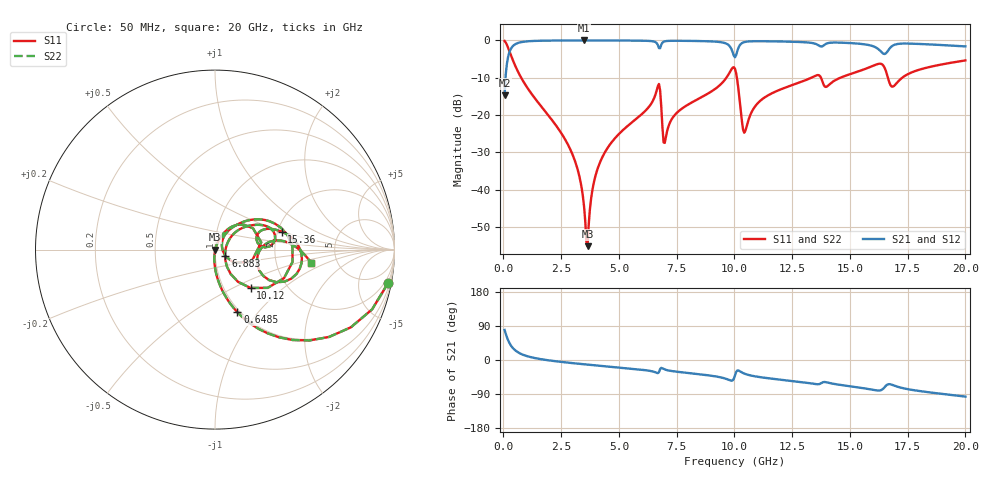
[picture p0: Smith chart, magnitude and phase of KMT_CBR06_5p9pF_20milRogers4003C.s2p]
! Data measured by Modelithics Inc. support@modelithics.com 813-866-6335
! KEMET CBR0603 5.9pF, Pad Width= 0.851mm, Pad Length= 0.64mm, Pad Gap= 0.62mm, 20mil Rogers 4003C substrate Data, January 2022
# hz S ma R 50
! 2 Port Network Data from SP1.SP block
! freq  magS11  angS11  magS21  angS21  magS12  angS12  magS22  angS22
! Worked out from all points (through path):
!   401 points, 50 MHz to 20 GHz, reference 50 ohm
!   highest |S21| = -0.01 dB at 3.491 GHz (marker M1); lowest = -14.7 dB at 50 MHz (marker M2)
!   group delay of S21, straight-line fit = 14.9 ps
!   lowest |S11| = -55.1 dB at 3.641 GHz (marker M3), VSWR 1.00, Z = 50.2 + j0.0524 ohm
!   |S11| at or under -10 dB: 767.8 MHz to 9.652 GHz (8.884 GHz wide, 171 % of centre); 10.11 GHz to 13.33 GHz (3.222 GHz wide, 27.5 % of centre); 13.75 GHz to 14.59 GHz (842.9 MHz wide, 5.95 % of centre)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
!   |S22| runs from -55.1 to -0.1 dB; largest |S21 - S12| = 0
!   S11 on the Smith chart (normalised r, x): 50 MHz: 1, -11; 648.5 MHz: 0.97, -0.79; 6.883 GHz: 1.12, -0.08; 10.12 GHz: 1.33, -0.62; 15.36 GHz: 2.10, +0.49; 20 GHz: 3.19, -0.66
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5e7  0.9829 -10.8  0.1838 79.2  0.1838 79.2  0.9829 -10.8
2.495e8  0.7293 -44.0  0.6835 46.0  0.6835 46.0  0.7293 -44.0
6.485e8  0.371 -70.3  0.9279 19.6  0.9279 19.6  0.371 -70.3
2.74325e9  0.04291 -94.9  0.9977 -6.7  0.9977 -6.7  0.04291 -94.9
3.391625e9  0.01031 -92.5  0.9984 -10.7  0.9984 -10.7  0.01031 -92.5
3.491375e9  0.005893 -86.7  0.9984 -11.3  0.9984 -11.3  0.005893 -86.7
3.641e9  0.001751 17.4  0.9983 -12.2  0.9983 -12.2  0.001751 17.4
3.94025e9  0.01356 69.4  0.9982 -13.9  0.9982 -13.9  0.01356 69.4
4.33925e9  0.02959 70.6  0.9977 -16.1  0.9977 -16.1  0.02959 70.6
6.73325e9  0.2607 8.9  0.7884 -32.1  0.7884 -32.1  0.2607 8.9
6.882875e9  0.06889 -32.1  0.9318 -22.1  0.9318 -22.1  0.06889 -32.1
7.0325e9  0.05095 40.8  0.9786 -25.9  0.9786 -25.9  0.05095 40.8
9.576125e9  0.294 35.1  0.9231 -48.5  0.9231 -48.5  0.294 35.1
1.0025e10  0.4162 -22.4  0.5953 -40.3  0.5953 -40.3  0.4162 -22.4
1.012475e10  0.2914 -47.2  0.7202 -27.7  0.7202 -27.7  0.2914 -47.2
1.047388e10  0.06144 9.0  0.9559 -36.9  0.9559 -36.9  0.06144 9.0
1.1222e10  0.1648 40.1  0.9754 -46.2  0.9754 -46.2  0.1648 40.1
1.336662e10  0.3204 23.5  0.9228 -62.2  0.9228 -62.2  0.3204 23.5
1.536162e10  0.3845 15.0  0.9052 -72.4  0.9052 -72.4  0.3845 15.0
1.630925e10  0.4877 -9.2  0.728 -80.2  0.728 -80.2  0.4877 -9.2
1.670825e10  0.2727 -25.2  0.7715 -63.7  0.7715 -63.7  0.2727 -25.2
2e10  0.5393 -7.8  0.8306 -96.6  0.8306 -96.6  0.5393 -7.8
